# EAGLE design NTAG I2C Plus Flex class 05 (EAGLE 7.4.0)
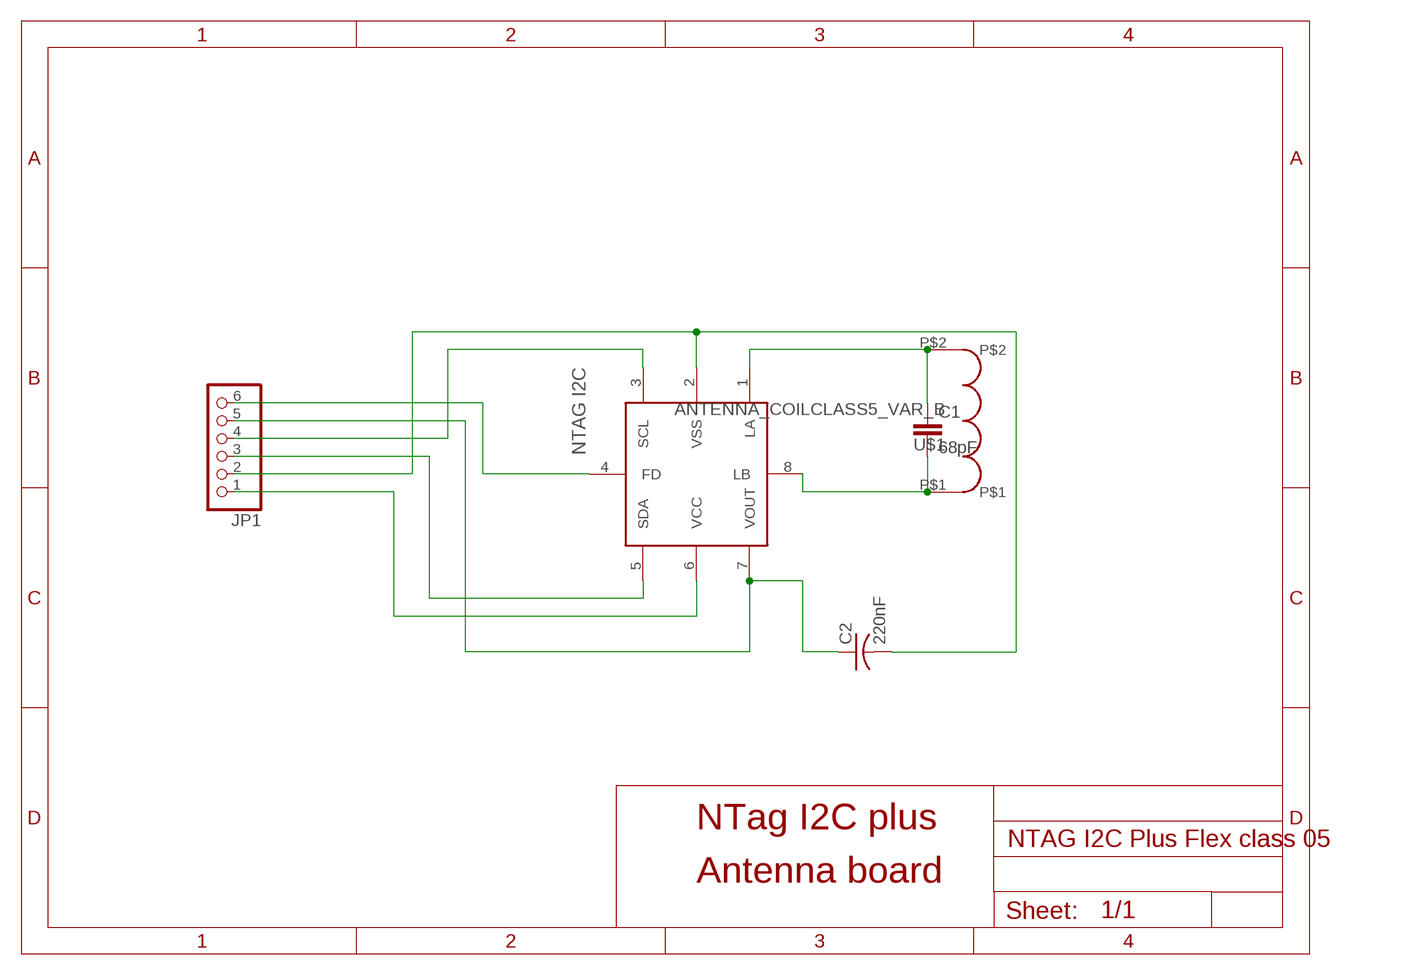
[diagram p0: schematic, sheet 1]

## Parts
C1  68pF  C-EUC0603  [C0603]
C2  220nF  C-USC0805  [C0805]
JP1  PINHD-1X6/90  [1X06/90]
NTAGUI  NTAG_I2C  [XQFN8]
U$1  ANTENNA_COILCLASS5_VAR_B  [L_PICC_50PF_CLASS5_B]

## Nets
+VCC: JP1.1 NTAGUI.6(VCC)
FD: JP1.6 NTAGUI.4(FD)
N$1: C1.1 NTAGUI.1(LA) U$1.P$2
N$2: C1.2 NTAGUI.8(LB) U$1.P$1
SCL: JP1.4 NTAGUI.3(SCL)
SDA: JP1.3 NTAGUI.5(SDA)
VOUT: C2.1 JP1.5 NTAGUI.7(VOUT)
VSS: C2.2 JP1.2 NTAGUI.2(VSS)

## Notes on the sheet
- NTag I2C plus
- Antenna board

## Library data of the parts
C1 = rcl:C-EU: CAPACITOR, European symbol
C2 = rcl:C-US: CAPACITOR, American symbol
JP1 = pinhead (2):PINHD-1X6: PIN HEADER
NTAGUI = NTAG I2C:NTAG_I2C
U$1 = NXP_PICC_Antennas:ANTENNA_COIL: Antenna coils designs for Class 4, Class 5 and Class 6

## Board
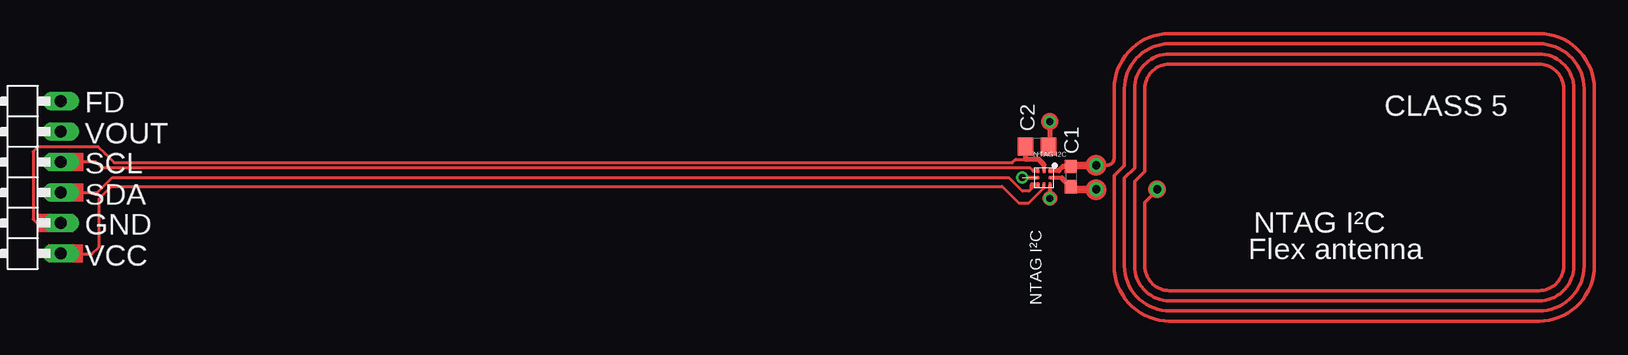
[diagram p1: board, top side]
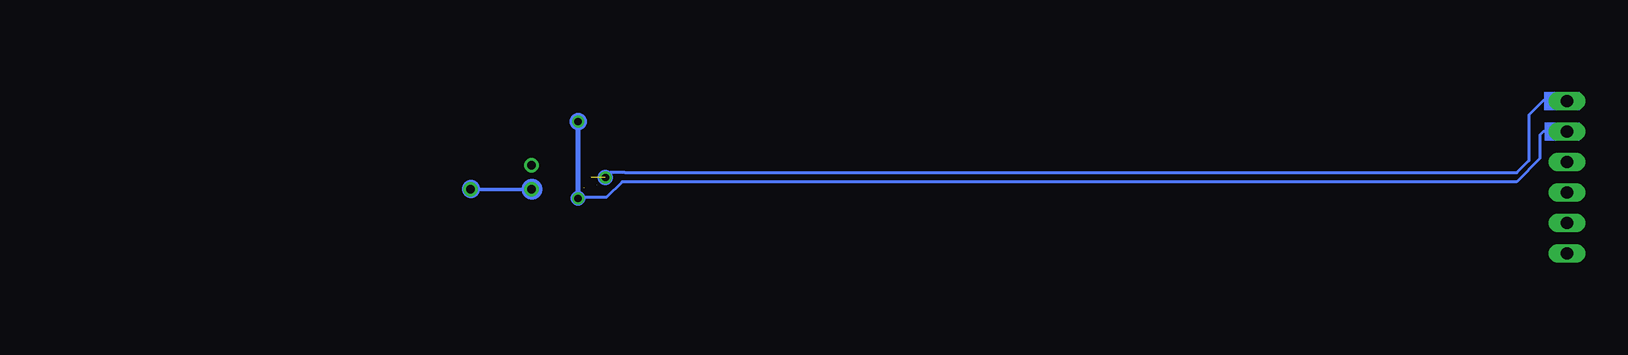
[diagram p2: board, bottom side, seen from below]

No outline drawn. Coordinates in mm, seen from the top.
Copper layers (1*16): Top 0.035mm / dielectric 1.5mm / Bottom 0.035mm
Design rules "default": minimum track width 10mil, minimum drill 24mil, track to track 8mil, track to pad 8mil, pad to pad 8mil, via to via 8mil, smd to smd 8mil, copper to edge 40mil, drill to drill 8mil, minimum pad ring 10mil, minimum via ring 8mil, stop-mask expansion 4mil, vias tented up to drill 0mil, thermal gap 10mil

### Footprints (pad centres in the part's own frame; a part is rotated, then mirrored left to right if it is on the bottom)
C0603 = smd 1.1 x 1: 1 -0.85,0; 2 0.85,0
C0805 = smd 1.3 x 1.5: 1 -0.95,0; 2 0.95,0
1X06/90 = drill 1.016 long: 1 -6.35,-3.81; 2 -3.81,-3.81; 3 -1.27,-3.81; 4 1.27,-3.81; 5 3.81,-3.81; 6 6.35,-3.81
XQFN8 = smd 0.4 x 0.32: 1 -0.6,0.55 | smd 0.4 x 0.22: 2 -0.6,0; 3 -0.6,-0.5; 5 0.6,-0.5; 6 0.6,0; 7 0.6,0.5 | smd 0.22 x 0.4: 4 0,-0.6; 8 0,0.6
L_PICC_50PF_CLASS5_B = drill 0.7: P$1 21.5,1; P$2 21.5,-1; P$3 16.42,1

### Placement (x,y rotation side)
C1  95.19,14.56 270 top
C2  92.36,17.09 180 top
JP1  7.2,14.5 90 top
NTAGUI  92.94,14.46 270 top
U$1  118.8,14.5 180 top

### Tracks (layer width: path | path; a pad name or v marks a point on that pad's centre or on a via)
+VCC  (1 unrouted)
  Top 0.254: JP1.1 11.06,8.1 13.6,8.1 14.2,8.7 14.2,12.72 15.23,13.75 89.46,13.75 90.89,12.33 91.64,12.33 92.94,13.63 | 92.94,13.64 NTAGUI.6
FD  (via drill 0.6)  (1 unrouted)
  Top 0.254: 92.3,14.5 NTAGUI.4 92.34,14.5
  Bottom 0.254: JP1.6 11.06,20.9 13,20.9 14.2,19.7 14.2,15.9 15.2,14.9 89.55,14.91 90.74,14.91 v91.14,14.5
N$1
  Top 0.254: 95.28,15.5 arc90 C1.1
  Top 0.406: C1.1 94.53,15.41 94.19,15.07 NTAGUI.1
  Top 0.61: U$1.P$2 95.19,15.5 C1.1
N$2
  Top 0.254: 94.44,14.46 NTAGUI.8
  Top 0.406: C1.2 94.44,14.46
  Top 0.61: U$1.P$1 95.19,13.5 C1.2
N$3
  Top 0.254: 92.45,14.5 91.2,14.5 | 91.15,14.5 91.2,14.5 | 91.2,14.5 91.2,14.45 92.45,14.45
N$7
  Top 0.254: 94.4,14.5 93.45,14.5 93.45,14.45 94.4,14.45
N$8
  Top 0.254: 92.95,15.3 92.95,15
N$9
  Top 0.254: 92,15.15 92.4,15.15 92.4,15 92.05,15 92.05,15.05
N$10
  Top 0.254: 91.9,13.9 91.9,13.95 92.45,13.95 92.45,13.75 92.05,13.75
N$11
  Top 0.254: 91.85,13.55 91.9,13.55 92.15,13.8 92.3,13.8
N$12
  Top 0.254: 92.95,13.95 92.95,13.85 92.95,13.65
N$13
  Top 0.254: 92.95,15.5 92.95,14.95
N$14
  Top 0.254: 93.45,13.95 93.45,13.25
SCL
  Top 0.254: JP1.4 13.95,15.77 14.44,15.28 91.79,15.28 92.01,15.06 NTAGUI.3
SDA  (1 unrouted)
  Top 0.254: JP1.3 13.28,13.23 13.29,13.22 14.05,13.22 15.31,14.49 90.01,14.49 91.15,13.35 91.71,13.35 91.85,13.49 91.85,13.86 | 91.85,13.86 NTAGUI.5
VOUT  (via drill 0.6)
  Top 0.254: v93.44,12.75 NTAGUI.7
  Top 0.406: v93.44,12.75 v93.43,12.75 | v93.43,19.15 93.43,17.09 C2.1
  Bottom 0.254: JP1.5 13.01,18.31 13.27,18.05 13.27,16.08 15.22,14.13 89.76,14.13 91.06,12.83 93.35,12.83 v93.43,12.75
  Bottom 0.406: v93.43,12.75 v93.43,19.15
VSS
  Top 0.254: JP1.2 9.01,10.69 8.7,11 8.7,16.65 9.1,17.05 14.15,17.05 14.7,16.5 14.7,16.48 15.46,15.72 90.32,15.72 90.6,16 91.4,16 | NTAGUI.2 92.94,15.57
  Top 0.406: C2.2 91.41,16.01 91.4,16 92.51,16 92.94,15.57
(copper drawn outside any net)
  shapes: Bottom area x2, Bottom circle x12, Top area x4, Top circle x23

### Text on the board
tNames: FD | CLASS 5 | VOUT | SCL | SDA | GND | NTAG I²C | Flex antenna | VCC | NTAG I²C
